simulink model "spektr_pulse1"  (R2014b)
settings: Solver=ode45  StartTime=0.0  StopTime=1  RelTol=1e-3
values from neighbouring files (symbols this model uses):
  f0 = 200    [mehrdeutigkeit_1.m]    (also in spektr_pulse_1.m = 1010; analog_filter_5.m = sqrt(fp1*fp2); impuls_antwort_1.m = sqrt(1/(L*C))/(2*pi); impuls_antwort_2.m = sqrt(1/(L*C))/(2*pi))
  N = 4*1024    (= 4096)    [ad_test_12.m]    (also in ad_test_2.m; ad_test_3.m; DA_wandler_spektr_1.m = 1000; DA_wandler_spektr_2.m = 1024)
  tast = 0.1    [fourier_reihe_DFT_1.m]    (also in fourier_reihe_rechteck_1.m; fourier_reihe_rechteck_2.m; spektr_pulse_1.m = 50)
  wp = sum(hanning(N).^2)    [mehrdeutigkeit_1.m]    (also in spektr_pulse_1.m)
undefined symbols (not defined in the file or in its folder): get
libraries: dspspect3 x1, dspsnks4 x1, dspsigops x1

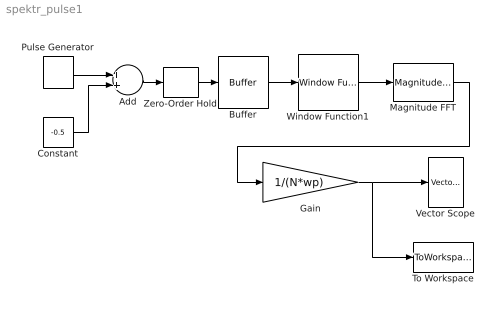
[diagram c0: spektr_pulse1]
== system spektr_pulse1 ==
  Add : Sum
  Buffer : Buffer  N=N  TreatMby1Signals=One channel
  Constant : Constant  Value=-0.5
  Gain : Gain  Gain=1/(N*wp)
  Magnitude FFT : dspspect3/Magnitude FFT  mag_or_magsq=Magnitude squared  FFTImplementation=Auto  fftLenInherit=on  fftsize=256  WrapInput=on
  Pulse Generator : DiscretePulseGenerator  PulseType=Time based  Period=1/f0  PulseWidth=tast
  To Workspace : ToWorkspace  VariableName=Y  SampleTime=-1
  Vector Scope : dspsnks4/Vector Scope  ScopeProperties=on  Domain=Frequency  HorizSpan=1  DisplayProperties=off  AxisGrid=on  Memory=off  FrameNumber=on  AxisLegend=off  AxisZoom=off  OpenScopeAtSimStart=on  OpenScopeImmediately=off  FigPos=get(0,'defaultfigureposition')  AxisProperties=off  XUnits=Hertz  XRange=[0...Fs]  InheritXIncr=on  XIncr=1/1024  XLabel=Time  XLimit=Auto  XMin=0  XMax=25000  XStart=0  YUnits=dB  YLabel=Leistung dB  LineProperties=off  XAxisParamsVer=6.9
  Window Function1 : dspsigops/Window Function  winmode=Apply window to input  wintype=Hanning  sampmode=Continuous  samptime=1  N=64  Rs=50  beta=10  winsamp=Symmetric  UserWindow=fenster  OptParams=off  UserParams={'symmetric'}  RowConvenienceOn=on  dataType=double  isSigned=on  wordLen=16  udDataType=sfix(16)  fracBitsMode=Best precision  numFracBits=15  roundingMode=Floor  overflowMode=off  numSidelobes=4  sidelobeLevel=-30
  Zero-Order Hold : ZeroOrderHold  SampleTime=1/(50000)
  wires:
  Zero-Order Hold/1 -> Buffer/1
  Magnitude FFT/1 -> Gain/1
  Gain/1 -> To Workspace/1, Vector Scope/1
  Buffer/1 -> Window Function1/1
  Add/1 -> Zero-Order Hold/1
  Pulse Generator/1 -> Add/1
  Constant/1 -> Add/2
  Window Function1/1 -> Magnitude FFT/1
